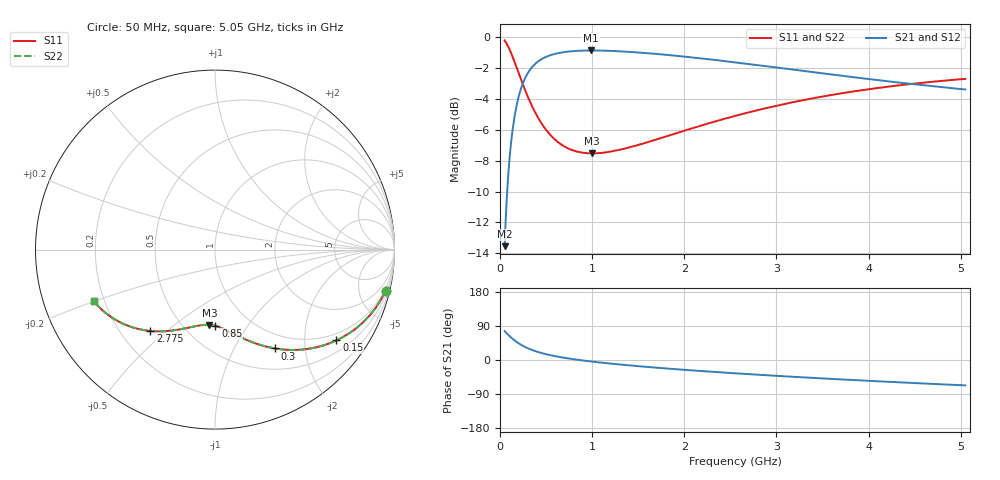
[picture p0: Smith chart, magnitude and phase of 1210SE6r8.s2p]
! AVX Thin Film Operation		Date: August 2001
! Description: Accu-P® Series, Thin Film, SMD, RF Capacitor
! Part Number: 12101J6R8BBT
! 50 MHz  -  5.05 GHz
! Serial Measurements
# mhz S db R 50
!	S11		S21		S12		S22
!	dB	Phase	dB	Phase	dB	Phase	dB	Phase
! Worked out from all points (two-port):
!   401 points, 50 MHz to 5.05 GHz, reference 50 ohm
!   highest |S21| = -0.85 dB at 987.5 MHz (marker M1); lowest = -13.5 dB at 50 MHz (marker M2)
!   |S21| within 3 dB of the highest: 202.2 MHz to end of sweep
!   lowest |S11| = -7.5 dB at 1 GHz (marker M3), VSWR 2.45, Z = 33.2 - j33.9 ohm
!   |S11| at or under -10 dB: nowhere
!   |S22| runs from -7.5 to -0.2 dB; largest |S21 - S12| = 0
!   S11 on the Smith chart (normalised r, x): 50 MHz: 0.80, -8.29; 150 MHz: 0.79, -2.81; 300 MHz: 0.78, -1.48; 850 MHz: 0.70, -0.72; 2.775 GHz: 0.32, -0.44; 5.05 GHz: 0.16, -0.20
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50  -0.20 -13.6  -13.54 76.4  -13.54 76.4  -0.20 -13.6
75  -0.43 -20.1  -10.28 69.9  -10.28 69.9  -0.43 -20.1
100  -0.73 -26.1  -8.12 63.9  -8.12 63.9  -0.73 -26.1
125  -1.08 -31.7  -6.58 58.3  -6.58 58.3  -1.08 -31.7
150  -1.46 -36.8  -5.44 53.2  -5.44 53.2  -1.46 -36.8
212.5  -2.48 -47.5  -3.62 42.5  -3.62 42.5  -2.48 -47.5
300  -3.82 -58.8  -2.33 31.2  -2.33 31.2  -3.82 -58.8
400  -5.07 -67.9  -1.62 22.1  -1.62 22.1  -5.07 -67.9
512.5  -6.09 -75.3  -1.23 14.6  -1.23 14.6  -6.09 -75.3
662.5  -6.94 -82.7  -0.98 7.3  -0.98 7.3  -6.94 -82.7
850  -7.42 -89.7  -0.87 0.3  -0.87 0.3  -7.42 -89.7
887.5  -7.47 -90.9  -0.86 -0.9  -0.86 -0.9  -7.47 -90.9
987.5  -7.52 -93.9  -0.85 -3.9  -0.85 -3.9  -7.52 -93.9
1000  -7.52 -94.2  -0.85 -4.3  -0.85 -4.3  -7.52 -94.2
1337.5  -7.24 -102.7  -0.91 -12.8  -0.91 -12.8  -7.24 -102.7
1725  -6.57 -110.8  -1.08 -20.8  -1.08 -20.8  -6.57 -110.8
2125  -5.82 -118.1  -1.32 -28.1  -1.32 -28.1  -5.82 -118.1
2550  -5.09 -125.1  -1.62 -35.1  -1.62 -35.1  -5.09 -125.1
2775  -4.75 -128.5  -1.78 -38.5  -1.78 -38.5  -4.75 -128.5
3387.5  -3.96 -137.1  -2.24 -47.2  -2.24 -47.2  -3.96 -137.1
4225  -3.18 -147.6  -2.86 -57.7  -2.86 -57.7  -3.18 -147.6
5050  -2.69 -157.0  -3.38 -67.0  -3.38 -67.0  -2.69 -157.0
